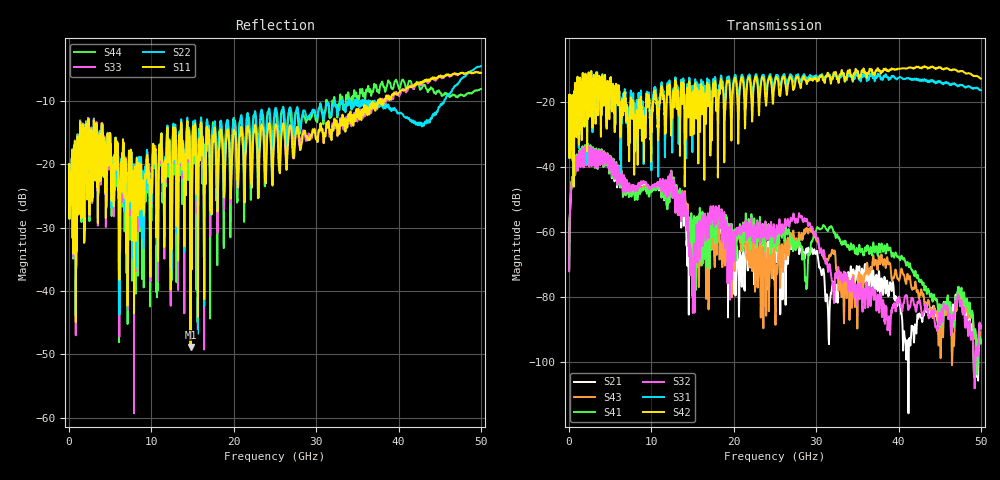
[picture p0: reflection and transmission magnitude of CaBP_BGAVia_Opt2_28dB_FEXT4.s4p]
!* Samtec Inc. NovaRay Examax Flyover System  *
!*  REV DATE  = 08/08/18  *
!*  TYPE  = TOUCHSTONE  *
!*  PORTS  = 4 port  *
!*  UNITS  = GHz  *
!*  DATA RANGE = DC  to 50 GHz; 10 MHz Step  *
!*  PARAMETER  = S  *
!*  FORMAT  = Real-Imaginary  *
!*  REFERENCE  = 50 ohms  *
!*  SOURCE  = HFSS  *
!*  VALIDATED  = No  *
!*  MANUFACTURER = SAMTEC  *
!*  INTERCONNECT = NVAx to EBCx to EBCx to NVAx  *
!*  [Full Channel NVAx to EBCx to EBCx to NVAx  with PCB Trace and BGA Via]  *
!*  BOUNDARY A  = Silicon BGA Ball Pad  *
!*  BOUNDARY B  = Silicon BGA Ball Pad  *
!*  NVAx (end a) ->>- (end b) NVAx  *
!*  Port 01 ->>- Port 02  *
!*  Port 03 ->>- Port 04  *
!***************************** CHANNEL MODEL ******************************************
# GHz S RI R 50
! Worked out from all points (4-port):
!   5000 points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, 10 MHz to 50 GHz, reference 50 ohm
!   strongest paths, dB at 10 MHz, 12.51 GHz, 25.01 GHz, 37.51 GHz, 50 GHz:
!     S42: -23.1, -23.5, -13.7, -9.7, -12.8
!     S31: -23.1, -28.5, -13.0, -11.3, -16.4
!     S32: -72.0, -45.4, -62.5, -79.5, -89.4
!     S41: -71.3, -44.5, -61.7, -66.8, -94.1
!     S43: -71.6, -44.7, -80.2, -70.6, -93.3
!     S21: -71.6, -45.4, -65.3, -76.7, -89.5
!   lowest |S11| = -48.8 dB at 14.75 GHz (marker M1), VSWR 1.01, Z = 49.7 - j0.221 ohm
!   |S11| at or under -10 dB: start of sweep to 37.51 GHz; 37.83997 GHz to 38.00552 GHz (165.6 MHz wide, 0.437 % of centre); 38.04261 GHz to 38.22467 GHz (182.1 MHz wide, 0.477 % of centre)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
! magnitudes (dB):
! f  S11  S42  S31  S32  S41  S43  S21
! 10 MHz  -22.1  -23.1  -23.1  -72.0  -71.3  -71.6  -71.6
! 780 MHz  -19.5  -16.9  -16.8  -41.0  -40.6  -40.7  -40.7
! 4.49 GHz  -22.8  -20.3  -20.9  -38.9  -39.0  -38.7  -39.3
! 12.53 GHz  -23.2  -24.8  -35.5  -45.1  -44.1  -44.4  -44.9
! 14.75 GHz  -48.8  -27.5  -22.0  -68.0  -64.3  -64.8  -61.4
! 28.08 GHz  -17.8  -15.4  -13.4  -55.1  -63.7  -61.3  -64.8
! 50 GHz  -5.6  -12.8  -16.4  -89.4  -94.1  -93.3  -89.5
